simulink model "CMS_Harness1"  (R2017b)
settings: Solver=FixedStepDiscrete  StartTime=0.0  StopTime=2  FixedStep=0.01  RelTol=1e-3  EnableMultiTasking=on
undefined symbols (not defined in the file): sigbuilder_block
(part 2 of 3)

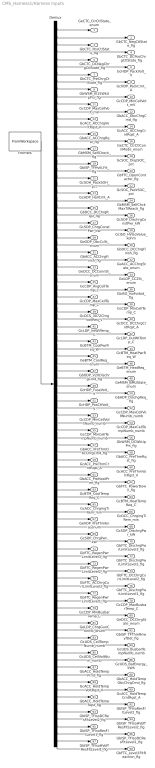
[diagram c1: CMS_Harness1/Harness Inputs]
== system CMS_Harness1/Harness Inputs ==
  Demux : Demux  Tag=STV Demux  Outputs=98
  FromWs : FromWorkspace  Tag=STV FromWs  VariableName=tuvar  SampleTime=0
  GeCTC_CtrCtlState_enum : Outport  Tag=STV Outport
  GbCTC_NegCtlState_flg : Outport  Tag=STV Outport  Port=2
  GbCTC_PosCtlState_flg : Outport  Tag=STV Outport  Port=3
  GbCTC_DCPosChrgCtlState_flg : Outport  Tag=STV Outport  Port=4
  GbCTC_DCNegChrgCtlState_flg : Outport  Tag=STV Outport  Port=5
  GcHDP_PackVolt_V : Outport  Tag=STV Outport  Port=6
  GbCTC_PreChrgCtlState_flg : Outport  Tag=STV Outport  Port=7
  GcHDP_PackCrnt_A : Outport  Tag=STV Outport  Port=8
  GbWSM_Kl15WkUpPrs_flg : Outport  Tag=STV Outport  Port=9
  GcCDP_MinCellVolt_mV : Outport  Tag=STV Outport  Port=10
  GcCDP_MaxCellVolt_mV : Outport  Tag=STV Outport  Port=11
  GbACC_ObcChrgCmd_flg : Outport  Tag=STV Outport  Port=12
  GcACC_ACChrgVoltRqst_V : Outport  Tag=STV Outport  Port=13
  GcACC_ACChrgCrntRqst_A : Outport  Tag=STV Outport  Port=14
  GbACC_ACChrgRqst_flg : Outport  Tag=STV Outport  Port=15
  GeCTC_CtrCtlConnMode_enum : Outport  Tag=STV Outport  Port=16
  GbMSM_SelfCheck_flg : Outport  Tag=STV Outport  Port=17
  GcSOC_DispSOC_pct : Outport  Tag=STV Outport  Port=18
  GbISP_TFHvilLFlt_flg : Outport  Tag=STV Outport  Port=19
  GbFTC_OpenContactor_flg : Outport  Tag=STV Outport  Port=20
  GcSOH_PackSOH_pct : Outport  Tag=STV Outport  Port=21
  GcSOC_PackSOC_pct : Outport  Tag=STV Outport  Port=22
  GcHDP_HallCrnt_A : Outport  Tag=STV Outport  Port=23
  GbMSM_SelfChckMaxTiReach_flg : Outport  Tag=STV Outport  Port=24
  GbDCC_DCChrgRqst_flg : Outport  Tag=STV Outport  Port=25
  GcSOP_DischrgConstPwr_kW : Outport  Tag=STV Outport  Port=26
  GcSOP_ChrgConstPwr_kW : Outport  Tag=STV Outport  Port=27
  GcISO_HVIsoValue_kohm : Outport  Tag=STV Outport  Port=28
  GeODP_ObcCcSt_enum : Outport  Tag=STV Outport  Port=29
  GbDCC_DCChrgFinish_flg : Outport  Tag=STV Outport  Port=30
  GbACC_ACChrgFinish_flg : Outport  Tag=STV Outport  Port=31
  GeACC_ACChrgState_enum : Outport  Tag=STV Outport  Port=32
  GeDCC_DCConnSt_enum : Outport  Tag=STV Outport  Port=33
  GeLDP_CC2St_enum : Outport  Tag=STV Outport  Port=34
  GcCDP_AvgCellTemp_C : Outport  Tag=STV Outport  Port=35
  GbISO_IsoForbid_flg : Outport  Tag=STV Outport  Port=36
  GcCDP_MaxCellTemp_C : Outport  Tag=STV Outport  Port=37
  GcCDP_MinCellTemp_C : Outport  Tag=STV Outport  Port=38
  GcDCS_3072ChrgVoltReq_V : Outport  Tag=STV Outport  Port=39
  GcDCC_DCChrgCrntRqst_A : Outport  Tag=STV Outport  Port=40
  GcLDP_lntWtTemp_C : Outport  Tag=STV Outport  Port=41
  GcLDP_OutWtTemp_C : Outport  Tag=STV Outport  Port=42
  GcBTM_CoolPwrReq_W : Outport  Tag=STV Outport  Port=43
  GcBTM_HeatPwrReq_W : Outport  Tag=STV Outport  Port=44
  GeBTM_CoolReq_enum : Outport  Tag=STV Outport  Port=45
  GeBTM_HeatReq_enum : Outport  Tag=STV Outport  Port=46
  GbODP_V2XDischrgCmd_flg : Outport  Tag=STV Outport  Port=47
  GeMSM_BMUState_enum : Outport  Tag=STV Outport  Port=48
  GcHDP_FuseVolt_V : Outport  Tag=STV Outport  Port=49
  GbADP_DischgReq_flg : Outport  Tag=STV Outport  Port=50
  GcHDP_PosCtlVolt_V : Outport  Tag=STV Outport  Port=51
  GcCDP_MaxCellVoltNumb_numb : Outport  Tag=STV Outport  Port=52
  GcCDP_MinCellVoltNumb_numb : Outport  Tag=STV Outport  Port=53
  GcCDP_MaxCellTempNumb_numb : Outport  Tag=STV Outport  Port=54
  GcCDP_MinCellTempNumb_numb : Outport  Tag=STV Outport  Port=55
  GbWSM_DCWkUpPrs_flg : Outport  Tag=STV Outport  Port=56
  GbACC_PreThmObcChrgCmd_flg : Outport  Tag=STV Outport  Port=57
  GbACC_PreThmRqst_flg : Outport  Tag=STV Outport  Port=58
  GcACC_PreThmCrntRqst_A : Outport  Tag=STV Outport  Port=59
  GcACC_PreThmVoltRqst_V : Outport  Tag=STV Outport  Port=60
  GbACC_PreHeatPrmt_flg : Outport  Tag=STV Outport  Port=61
  GbFTC_PowerDown_flg : Outport  Tag=STV Outport  Port=62
  GcBTM_CoolTempReq_C : Outport  Tag=STV Outport  Port=63
  GcBTM_HeatTempReq_C : Outport  Tag=STV Outport  Port=64
  GcACC_ChrgingTiRem_min : Outport  Tag=STV Outport  Port=65
  GcDCC_ChrgingTiRem_min : Outport  Tag=STV Outport  Port=66
  GeVDP_PreThmEna_enum : Outport  Tag=STV Outport  Port=67
  GcSOP_DischrgPwr_kW : Outport  Tag=STV Outport  Port=68
  GcSOP_ChrgPwr_kW : Outport  Tag=STV Outport  Port=69
  GbFTC_DischrgPwrLimitLevel3_flg : Outport  Tag=STV Outport  Port=70
  GbFTC_RegenPwrLimitLevel3_flg : Outport  Tag=STV Outport  Port=71
  GbFTC_DischrgPwrLimitLevel2_flg : Outport  Tag=STV Outport  Port=72
  GbFTC_RegenPwrLimitLevel2_flg : Outport  Tag=STV Outport  Port=73
  GbFTC_DCChrgCurrLimitLevel2_flg : Outport  Tag=STV Outport  Port=74
  GbFTC_ACChrgCurrLimitLevel2_flg : Outport  Tag=STV Outport  Port=75
  GbFTC_DischrgPwrLimitLevel1_flg : Outport  Tag=STV Outport  Port=76
  GbFTC_RegenPwrLimitLevel1_flg : Outport  Tag=STV Outport  Port=77
  GcCDP_MaxBusbarTemp_C : Outport  Tag=STV Outport  Port=78
  GcCDP_MinBusbarTemp_C : Outport  Tag=STV Outport  Port=79
  GeDCC_DCChrgState_enum : Outport  Tag=STV Outport  Port=80
  GeLDP_ChrgGunConnSt_enum : Outport  Tag=STV Outport  Port=81
  GbISP_TFThmRnwyfDet_flg : Outport  Tag=STV Outport  Port=82
  GcUDS_CellTempNumb_numb : Outport  Tag=STV Outport  Port=83
  GcUDS_BusbarTempNumb_numb : Outport  Tag=STV Outport  Port=84
  GcUDS_CellVoltNum_numb : Outport  Tag=STV Outport  Port=85
  GcUDS_BatEnergy_kWh : Outport  Tag=STV Outport  Port=86
  GbACC_HoldTempPrmt_flg : Outport  Tag=STV Outport  Port=87
  GbACC_HoldTempObcChrgCmd_flg : Outport  Tag=STV Outport  Port=88
  GcACC_HoldTempVoltRqst_V : Outport  Tag=STV Outport  Port=89
  GcACC_HoldTempCrntRqst_A : Outport  Tag=STV Outport  Port=90
  GbACC_HoldTempRqst_flg : Outport  Tag=STV Outport  Port=91
  GbISP_TFIsoResFltLevel2_flg : Outport  Tag=STV Outport  Port=92
  GbISP_TFIsoDCResFltLevel2_flg : Outport  Tag=STV Outport  Port=93
  GbISP_TFIsoHVoffResFltLevel2_flg : Outport  Tag=STV Outport  Port=94
  GbISP_TFIsoResFltLevel1_flg : Outport  Tag=STV Outport  Port=95
  GbISP_TFIsoDCResFltLevel1_flg : Outport  Tag=STV Outport  Port=96
  GbISP_TFIsoHVoffResFltLevel1_flg : Outport  Tag=STV Outport  Port=97
  GbFTC_Level1FltReaction_flg : Outport  Tag=STV Outport  Port=98
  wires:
  FromWs/1 -> Demux/1
  Demux/1 -> GeCTC_CtrCtlState_enum/1
  Demux/2 -> GbCTC_NegCtlState_flg/1
  Demux/3 -> GbCTC_PosCtlState_flg/1
  Demux/4 -> GbCTC_DCPosChrgCtlState_flg/1
  Demux/5 -> GbCTC_DCNegChrgCtlState_flg/1
  Demux/6 -> GcHDP_PackVolt_V/1
  Demux/7 -> GbCTC_PreChrgCtlState_flg/1
  Demux/8 -> GcHDP_PackCrnt_A/1
  Demux/9 -> GbWSM_Kl15WkUpPrs_flg/1
  Demux/10 -> GcCDP_MinCellVolt_mV/1
  Demux/11 -> GcCDP_MaxCellVolt_mV/1
  Demux/12 -> GbACC_ObcChrgCmd_flg/1
  Demux/13 -> GcACC_ACChrgVoltRqst_V/1
  Demux/14 -> GcACC_ACChrgCrntRqst_A/1
  Demux/15 -> GbACC_ACChrgRqst_flg/1
  Demux/16 -> GeCTC_CtrCtlConnMode_enum/1
  Demux/17 -> GbMSM_SelfCheck_flg/1
  Demux/18 -> GcSOC_DispSOC_pct/1
  Demux/19 -> GbISP_TFHvilLFlt_flg/1
  Demux/20 -> GbFTC_OpenContactor_flg/1
  Demux/21 -> GcSOH_PackSOH_pct/1
  Demux/22 -> GcSOC_PackSOC_pct/1
  Demux/23 -> GcHDP_HallCrnt_A/1
  Demux/24 -> GbMSM_SelfChckMaxTiReach_flg/1
  Demux/25 -> GbDCC_DCChrgRqst_flg/1
  Demux/26 -> GcSOP_DischrgConstPwr_kW/1
  Demux/27 -> GcSOP_ChrgConstPwr_kW/1
  Demux/28 -> GcISO_HVIsoValue_kohm/1
  Demux/29 -> GeODP_ObcCcSt_enum/1
  Demux/30 -> GbDCC_DCChrgFinish_flg/1
  Demux/31 -> GbACC_ACChrgFinish_flg/1
  Demux/32 -> GeACC_ACChrgState_enum/1
  Demux/33 -> GeDCC_DCConnSt_enum/1
  Demux/34 -> GeLDP_CC2St_enum/1
  Demux/35 -> GcCDP_AvgCellTemp_C/1
  Demux/36 -> GbISO_IsoForbid_flg/1
  Demux/37 -> GcCDP_MaxCellTemp_C/1
  Demux/38 -> GcCDP_MinCellTemp_C/1
  Demux/39 -> GcDCS_3072ChrgVoltReq_V/1
  Demux/40 -> GcDCC_DCChrgCrntRqst_A/1
  Demux/41 -> GcLDP_lntWtTemp_C/1
  Demux/42 -> GcLDP_OutWtTemp_C/1
  Demux/43 -> GcBTM_CoolPwrReq_W/1
  Demux/44 -> GcBTM_HeatPwrReq_W/1
  Demux/45 -> GeBTM_CoolReq_enum/1
  Demux/46 -> GeBTM_HeatReq_enum/1
  Demux/47 -> GbODP_V2XDischrgCmd_flg/1
  Demux/48 -> GeMSM_BMUState_enum/1
  Demux/49 -> GcHDP_FuseVolt_V/1
  Demux/50 -> GbADP_DischgReq_flg/1
  Demux/51 -> GcHDP_PosCtlVolt_V/1
  Demux/52 -> GcCDP_MaxCellVoltNumb_numb/1
  Demux/53 -> GcCDP_MinCellVoltNumb_numb/1
  Demux/54 -> GcCDP_MaxCellTempNumb_numb/1
  Demux/55 -> GcCDP_MinCellTempNumb_numb/1
  Demux/56 -> GbWSM_DCWkUpPrs_flg/1
  Demux/57 -> GbACC_PreThmObcChrgCmd_flg/1
  Demux/58 -> GbACC_PreThmRqst_flg/1
  Demux/59 -> GcACC_PreThmCrntRqst_A/1
  Demux/60 -> GcACC_PreThmVoltRqst_V/1
  Demux/61 -> GbACC_PreHeatPrmt_flg/1
  Demux/62 -> GbFTC_PowerDown_flg/1
  Demux/63 -> GcBTM_CoolTempReq_C/1
  Demux/64 -> GcBTM_HeatTempReq_C/1
  Demux/65 -> GcACC_ChrgingTiRem_min/1
  Demux/66 -> GcDCC_ChrgingTiRem_min/1
  Demux/67 -> GeVDP_PreThmEna_enum/1
  Demux/68 -> GcSOP_DischrgPwr_kW/1
  Demux/69 -> GcSOP_ChrgPwr_kW/1
  Demux/70 -> GbFTC_DischrgPwrLimitLevel3_flg/1
  Demux/71 -> GbFTC_RegenPwrLimitLevel3_flg/1
  Demux/72 -> GbFTC_DischrgPwrLimitLevel2_flg/1
  Demux/73 -> GbFTC_RegenPwrLimitLevel2_flg/1
  Demux/74 -> GbFTC_DCChrgCurrLimitLevel2_flg/1
  Demux/75 -> GbFTC_ACChrgCurrLimitLevel2_flg/1
  Demux/76 -> GbFTC_DischrgPwrLimitLevel1_flg/1
  Demux/77 -> GbFTC_RegenPwrLimitLevel1_flg/1
  Demux/78 -> GcCDP_MaxBusbarTemp_C/1
  Demux/79 -> GcCDP_MinBusbarTemp_C/1
  Demux/80 -> GeDCC_DCChrgState_enum/1
  Demux/81 -> GeLDP_ChrgGunConnSt_enum/1
  Demux/82 -> GbISP_TFThmRnwyfDet_flg/1
  Demux/83 -> GcUDS_CellTempNumb_numb/1
  Demux/84 -> GcUDS_BusbarTempNumb_numb/1
  Demux/85 -> GcUDS_CellVoltNum_numb/1
  Demux/86 -> GcUDS_BatEnergy_kWh/1
  Demux/87 -> GbACC_HoldTempPrmt_flg/1
  Demux/88 -> GbACC_HoldTempObcChrgCmd_flg/1
  Demux/89 -> GcACC_HoldTempVoltRqst_V/1
  Demux/90 -> GcACC_HoldTempCrntRqst_A/1
  Demux/91 -> GbACC_HoldTempRqst_flg/1
  Demux/92 -> GbISP_TFIsoResFltLevel2_flg/1
  Demux/93 -> GbISP_TFIsoDCResFltLevel2_flg/1
  Demux/94 -> GbISP_TFIsoHVoffResFltLevel2_flg/1
  Demux/95 -> GbISP_TFIsoResFltLevel1_flg/1
  Demux/96 -> GbISP_TFIsoDCResFltLevel1_flg/1
  Demux/97 -> GbISP_TFIsoHVoffResFltLevel1_flg/1
  Demux/98 -> GbFTC_Level1FltReaction_flg/1

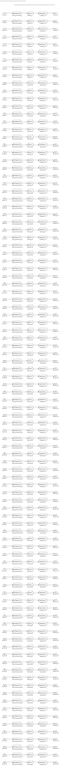
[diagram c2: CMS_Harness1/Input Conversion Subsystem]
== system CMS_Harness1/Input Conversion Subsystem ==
  note: This subsystem has been inserted by Simulink to adapt the output of the source blocks to the interface required by the harnessed component. Modifying the contents of this subsystem may result in compilation and simulation failure.
  Inport_1 : Inport
  Inport_2 : Inport  Port=2
  Inport_3 : Inport  Port=3
  Inport_4 : Inport  Port=4
  Inport_5 : Inport  Port=5
  Inport_6 : Inport  Port=6
  Inport_7 : Inport  Port=7
  Inport_8 : Inport  Port=8
  Inport_9 : Inport  Port=9
  Inport_10 : Inport  Port=10
  Inport_11 : Inport  Port=11
  Inport_12 : Inport  Port=12
  Inport_13 : Inport  Port=13
  Inport_14 : Inport  Port=14
  Inport_15 : Inport  Port=15
  Inport_16 : Inport  Port=16
  Inport_17 : Inport  Port=17
  Inport_18 : Inport  Port=18
  Inport_19 : Inport  Port=19
  Inport_20 : Inport  Port=20
  Inport_21 : Inport  Port=21
  Inport_22 : Inport  Port=22
  Inport_23 : Inport  Port=23
  Inport_24 : Inport  Port=24
  Inport_25 : Inport  Port=25
  Inport_26 : Inport  Port=26
  Inport_27 : Inport  Port=27
  Inport_28 : Inport  Port=28
  Inport_29 : Inport  Port=29
  Inport_30 : Inport  Port=30
  Inport_31 : Inport  Port=31
  Inport_32 : Inport  Port=32
  Inport_33 : Inport  Port=33
  Inport_34 : Inport  Port=34
  Inport_35 : Inport  Port=35
  Inport_36 : Inport  Port=36
  Inport_37 : Inport  Port=37
  Inport_38 : Inport  Port=38
  Inport_39 : Inport  Port=39
  Inport_40 : Inport  Port=40
  Inport_41 : Inport  Port=41
  Inport_42 : Inport  Port=42
  Inport_43 : Inport  Port=43
  Inport_44 : Inport  Port=44
  Inport_45 : Inport  Port=45
  Inport_46 : Inport  Port=46
  Inport_47 : Inport  Port=47
  Inport_48 : Inport  Port=48
  Inport_49 : Inport  Port=49
  Inport_50 : Inport  Port=50
  Inport_51 : Inport  Port=51
  Inport_52 : Inport  Port=52
  Inport_53 : Inport  Port=53
  Inport_54 : Inport  Port=54
  Inport_55 : Inport  Port=55
  Inport_56 : Inport  Port=56
  Inport_57 : Inport  Port=57
  Inport_58 : Inport  Port=58
  Inport_59 : Inport  Port=59
  Inport_60 : Inport  Port=60
  Inport_61 : Inport  Port=61
  Inport_62 : Inport  Port=62
  Inport_63 : Inport  Port=63
  Inport_64 : Inport  Port=64
  Inport_65 : Inport  Port=65
  Inport_66 : Inport  Port=66
  Inport_67 : Inport  Port=67
  Inport_68 : Inport  Port=68
  Inport_69 : Inport  Port=69
  Inport_70 : Inport  Port=70
  Inport_71 : Inport  Port=71
  Inport_72 : Inport  Port=72
  Inport_73 : Inport  Port=73
  Inport_74 : Inport  Port=74
  Inport_75 : Inport  Port=75
  Inport_76 : Inport  Port=76
  Inport_77 : Inport  Port=77
  Inport_78 : Inport  Port=78
  Inport_79 : Inport  Port=79
  Inport_80 : Inport  Port=80
  Inport_81 : Inport  Port=81
  Inport_82 : Inport  Port=82
  Inport_83 : Inport  Port=83
  Inport_84 : Inport  Port=84
  Inport_85 : Inport  Port=85
  Inport_86 : Inport  Port=86
  Inport_87 : Inport  Port=87
  Inport_88 : Inport  Port=88
  Inport_89 : Inport  Port=89
  Inport_90 : Inport  Port=90
  Inport_91 : Inport  Port=91
  Inport_92 : Inport  Port=92
  Inport_93 : Inport  Port=93
  Inport_94 : Inport  Port=94
  Inport_95 : Inport  Port=95
  Inport_96 : Inport  Port=96
  Inport_97 : Inport  Port=97
  Inport_98 : Inport  Port=98
  Data_Conversion_{1,16,29,32..34,45..46,48,52..55,67,80..81,83..85} (19 alike) : DataTypeConversion  OutDataTypeStr=uint8
  Data_Conversion_{10..11,28,65..66,86} (6 alike) : DataTypeConversion  OutDataTypeStr=uint16
  Data_Conversion_{2..5,7,9,12,15,17,19..20,24..25,30..31,36,47,50,56..58,61..62,70..77,82,87..88,91..98} (42 alike) : DataTypeConversion  OutDataTypeStr=boolean
  Data_Conversion_{6,8,13..14,18,21..23,26..27,35,37..38,40..44,49,51,59..60,63..64,68..69,78..79,89..90} (30 alike) : DataTypeConversion  OutDataTypeStr=single
  Data_Conversion_39 : DataTypeConversion  OutDataTypeStr=fixdt('ufix16_Sp1')
  RateTs_{1..98} (98 alike) : RateTransition  OutPortSampleTime=0.01
  SigSpec_{1,16,32..34,45..46,48,67,80} (10 alike) : SignalSpecification  OutDataTypeStr=uint8  Unit=enum  Dimensions=[1]  SampleTime=0.01
  SigSpec_10 : SignalSpecification  OutDataTypeStr=uint16  Unit=mV  Dimensions=[1]  SampleTime=0.01
  SigSpec_11 : SignalSpecification  OutDataTypeStr=uint16  Unit=mV  Dimensions=[1]  SampleTime=0.01
  SigSpec_{12,15,17,19..20,24..25,30..31,36,47,57..58,61..62,70..77,82,87..88,91..98} (34 alike) : SignalSpecification  OutDataTypeStr=boolean  Unit=flag  Dimensions=[1]  SampleTime=0.01
  SigSpec_{6,13,49,51,60,89} (6 alike) : SignalSpecification  OutDataTypeStr=single  Unit=V  Dimensions=[1]  SampleTime=0.01
  SigSpec_{8,14,23,40,59,90} (6 alike) : SignalSpecification  OutDataTypeStr=single  Unit=A  Dimensions=[1]  SampleTime=0.01
  SigSpec_18 : SignalSpecification  OutDataTypeStr=single  Unit=pct  Dimensions=[1]  SampleTime=0.01
  SigSpec_{2..5,7,9,50,56} (8 alike) : SignalSpecification  OutDataTypeStr=boolean  Unit=flg  Dimensions=[1]  SampleTime=0.01
  SigSpec_21 : SignalSpecification  OutDataTypeStr=single  Unit=pct  Dimensions=[1]  SampleTime=0.01
  SigSpec_22 : SignalSpecification  OutDataTypeStr=single  Unit=pct  Dimensions=[1]  SampleTime=0.01
  SigSpec_{26..27,68..69} (4 alike) : SignalSpecification  OutDataTypeStr=single  Unit=kW  Dimensions=[1]  SampleTime=0.01
  SigSpec_28 : SignalSpecification  OutDataTypeStr=uint16  Unit=kohm  Dimensions=[1]  SampleTime=0.01
  SigSpec_{29,52..55,81,83..85} (9 alike) : SignalSpecification  OutDataTypeStr=uint8  Unit=numb  Dimensions=[1]  SampleTime=0.01
  SigSpec_{35,37..38,41..42,63..64,78..79} (9 alike) : SignalSpecification  OutDataTypeStr=single  Unit=C  Dimensions=[1]  SampleTime=0.01
  SigSpec_39 : SignalSpecification  OutDataTypeStr=fixdt('ufix16_Sp1')  Unit=V  Dimensions=[1]  SampleTime=0.01
  SigSpec_43 : SignalSpecification  OutDataTypeStr=single  Unit=W  Dimensions=[1]  SampleTime=0.01
  SigSpec_44 : SignalSpecification  OutDataTypeStr=single  Unit=W  Dimensions=[1]  SampleTime=0.01
  SigSpec_65 : SignalSpecification  OutDataTypeStr=uint16  Unit=min  Dimensions=[1]  SampleTime=0.01
  SigSpec_66 : SignalSpecification  OutDataTypeStr=uint16  Unit=min  Dimensions=[1]  SampleTime=0.01
  SigSpec_86 : SignalSpecification  OutDataTypeStr=uint16  Unit=kWh  Dimensions=[1]  SampleTime=0.01
  Outport_1 : Outport
  Outport_2 : Outport  Port=2
  Outport_3 : Outport  Port=3
  Outport_4 : Outport  Port=4
  Outport_5 : Outport  Port=5
  Outport_6 : Outport  Port=6
  Outport_7 : Outport  Port=7
  Outport_8 : Outport  Port=8
  Outport_9 : Outport  Port=9
  Outport_10 : Outport  Port=10
  Outport_11 : Outport  Port=11
  Outport_12 : Outport  Port=12
  Outport_13 : Outport  Port=13
  Outport_14 : Outport  Port=14
  Outport_15 : Outport  Port=15
  Outport_16 : Outport  Port=16
  Outport_17 : Outport  Port=17
  Outport_18 : Outport  Port=18
  Outport_19 : Outport  Port=19
  Outport_20 : Outport  Port=20
  Outport_21 : Outport  Port=21
  Outport_22 : Outport  Port=22
  Outport_23 : Outport  Port=23
  Outport_24 : Outport  Port=24
  Outport_25 : Outport  Port=25
  Outport_26 : Outport  Port=26
  Outport_27 : Outport  Port=27
  Outport_28 : Outport  Port=28
  Outport_29 : Outport  Port=29
  Outport_30 : Outport  Port=30
  Outport_31 : Outport  Port=31
  Outport_32 : Outport  Port=32
  Outport_33 : Outport  Port=33
  Outport_34 : Outport  Port=34
  Outport_35 : Outport  Port=35
  Outport_36 : Outport  Port=36
  Outport_37 : Outport  Port=37
  Outport_38 : Outport  Port=38
  Outport_39 : Outport  Port=39
  Outport_40 : Outport  Port=40
  Outport_41 : Outport  Port=41
  Outport_42 : Outport  Port=42
  Outport_43 : Outport  Port=43
  Outport_44 : Outport  Port=44
  Outport_45 : Outport  Port=45
  Outport_46 : Outport  Port=46
  Outport_47 : Outport  Port=47
  Outport_48 : Outport  Port=48
  Outport_49 : Outport  Port=49
  Outport_50 : Outport  Port=50
  Outport_51 : Outport  Port=51
  Outport_52 : Outport  Port=52
  Outport_53 : Outport  Port=53
  Outport_54 : Outport  Port=54
  Outport_55 : Outport  Port=55
  Outport_56 : Outport  Port=56
  Outport_57 : Outport  Port=57
  Outport_58 : Outport  Port=58
  Outport_59 : Outport  Port=59
  Outport_60 : Outport  Port=60
  Outport_61 : Outport  Port=61
  Outport_62 : Outport  Port=62
  Outport_63 : Outport  Port=63
  Outport_64 : Outport  Port=64
  Outport_65 : Outport  Port=65
  Outport_66 : Outport  Port=66
  Outport_67 : Outport  Port=67
  Outport_68 : Outport  Port=68
  Outport_69 : Outport  Port=69
  Outport_70 : Outport  Port=70
  Outport_71 : Outport  Port=71
  Outport_72 : Outport  Port=72
  Outport_73 : Outport  Port=73
  Outport_74 : Outport  Port=74
  Outport_75 : Outport  Port=75
  Outport_76 : Outport  Port=76
  Outport_77 : Outport  Port=77
  Outport_78 : Outport  Port=78
  Outport_79 : Outport  Port=79
  Outport_80 : Outport  Port=80
  Outport_81 : Outport  Port=81
  Outport_82 : Outport  Port=82
  Outport_83 : Outport  Port=83
  Outport_84 : Outport  Port=84
  Outport_85 : Outport  Port=85
  Outport_86 : Outport  Port=86
  Outport_87 : Outport  Port=87
  Outport_88 : Outport  Port=88
  Outport_89 : Outport  Port=89
  Outport_90 : Outport  Port=90
  Outport_91 : Outport  Port=91
  Outport_92 : Outport  Port=92
  Outport_93 : Outport  Port=93
  Outport_94 : Outport  Port=94
  Outport_95 : Outport  Port=95
  Outport_96 : Outport  Port=96
  Outport_97 : Outport  Port=97
  Outport_98 : Outport  Port=98
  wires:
  SigSpec_1/1 -> Outport_1/1
  RateTs_1/1 -> SigSpec_1/1
  Data_Conversion_1/1 -> RateTs_1/1
  Inport_1/1 -> Data_Conversion_1/1
  SigSpec_2/1 -> Outport_2/1
  RateTs_2/1 -> SigSpec_2/1
  Data_Conversion_2/1 -> RateTs_2/1
  Inport_2/1 -> Data_Conversion_2/1
  SigSpec_3/1 -> Outport_3/1
  RateTs_3/1 -> SigSpec_3/1
  Data_Conversion_3/1 -> RateTs_3/1
  Inport_3/1 -> Data_Conversion_3/1
  SigSpec_4/1 -> Outport_4/1
  RateTs_4/1 -> SigSpec_4/1
  Data_Conversion_4/1 -> RateTs_4/1
  Inport_4/1 -> Data_Conversion_4/1
  SigSpec_5/1 -> Outport_5/1
  RateTs_5/1 -> SigSpec_5/1
  Data_Conversion_5/1 -> RateTs_5/1
  Inport_5/1 -> Data_Conversion_5/1
  SigSpec_6/1 -> Outport_6/1
  RateTs_6/1 -> SigSpec_6/1
  Data_Conversion_6/1 -> RateTs_6/1
  Inport_6/1 -> Data_Conversion_6/1
  SigSpec_7/1 -> Outport_7/1
  RateTs_7/1 -> SigSpec_7/1
  Data_Conversion_7/1 -> RateTs_7/1
  Inport_7/1 -> Data_Conversion_7/1
  SigSpec_8/1 -> Outport_8/1
  RateTs_8/1 -> SigSpec_8/1
  Data_Conversion_8/1 -> RateTs_8/1
  Inport_8/1 -> Data_Conversion_8/1
  SigSpec_9/1 -> Outport_9/1
  RateTs_9/1 -> SigSpec_9/1
  Data_Conversion_9/1 -> RateTs_9/1
  Inport_9/1 -> Data_Conversion_9/1
  SigSpec_10/1 -> Outport_10/1
  RateTs_10/1 -> SigSpec_10/1
  Data_Conversion_10/1 -> RateTs_10/1
  Inport_10/1 -> Data_Conversion_10/1
  SigSpec_11/1 -> Outport_11/1
  RateTs_11/1 -> SigSpec_11/1
  Data_Conversion_11/1 -> RateTs_11/1
  Inport_11/1 -> Data_Conversion_11/1
  SigSpec_12/1 -> Outport_12/1
  RateTs_12/1 -> SigSpec_12/1
  Data_Conversion_12/1 -> RateTs_12/1
  Inport_12/1 -> Data_Conversion_12/1
  SigSpec_13/1 -> Outport_13/1
  RateTs_13/1 -> SigSpec_13/1
  Data_Conversion_13/1 -> RateTs_13/1
  Inport_13/1 -> Data_Conversion_13/1
  SigSpec_14/1 -> Outport_14/1
  RateTs_14/1 -> SigSpec_14/1
  Data_Conversion_14/1 -> RateTs_14/1
  Inport_14/1 -> Data_Conversion_14/1
  SigSpec_15/1 -> Outport_15/1
  RateTs_15/1 -> SigSpec_15/1
  Data_Conversion_15/1 -> RateTs_15/1
  Inport_15/1 -> Data_Conversion_15/1
  SigSpec_16/1 -> Outport_16/1
  RateTs_16/1 -> SigSpec_16/1
  Data_Conversion_16/1 -> RateTs_16/1
  Inport_16/1 -> Data_Conversion_16/1
  SigSpec_17/1 -> Outport_17/1
  RateTs_17/1 -> SigSpec_17/1
  Data_Conversion_17/1 -> RateTs_17/1
  Inport_17/1 -> Data_Conversion_17/1
  SigSpec_18/1 -> Outport_18/1
  RateTs_18/1 -> SigSpec_18/1
  Data_Conversion_18/1 -> RateTs_18/1
  Inport_18/1 -> Data_Conversion_18/1
  SigSpec_19/1 -> Outport_19/1
  RateTs_19/1 -> SigSpec_19/1
  Data_Conversion_19/1 -> RateTs_19/1
  Inport_19/1 -> Data_Conversion_19/1
  SigSpec_20/1 -> Outport_20/1
  RateTs_20/1 -> SigSpec_20/1
  Data_Conversion_20/1 -> RateTs_20/1
  Inport_20/1 -> Data_Conversion_20/1
  SigSpec_21/1 -> Outport_21/1
  RateTs_21/1 -> SigSpec_21/1
  Data_Conversion_21/1 -> RateTs_21/1
  Inport_21/1 -> Data_Conversion_21/1
  SigSpec_22/1 -> Outport_22/1
  RateTs_22/1 -> SigSpec_22/1
  Data_Conversion_22/1 -> RateTs_22/1
  Inport_22/1 -> Data_Conversion_22/1
  SigSpec_23/1 -> Outport_23/1
  RateTs_23/1 -> SigSpec_23/1
  Data_Conversion_23/1 -> RateTs_23/1
  Inport_23/1 -> Data_Conversion_23/1
  SigSpec_24/1 -> Outport_24/1
  RateTs_24/1 -> SigSpec_24/1
  Data_Conversion_24/1 -> RateTs_24/1
  Inport_24/1 -> Data_Conversion_24/1
  SigSpec_25/1 -> Outport_25/1
  RateTs_25/1 -> SigSpec_25/1
  Data_Conversion_25/1 -> RateTs_25/1
  Inport_25/1 -> Data_Conversion_25/1
  SigSpec_26/1 -> Outport_26/1
  RateTs_26/1 -> SigSpec_26/1
  Data_Conversion_26/1 -> RateTs_26/1
  Inport_26/1 -> Data_Conversion_26/1
  SigSpec_27/1 -> Outport_27/1
  RateTs_27/1 -> SigSpec_27/1
  Data_Conversion_27/1 -> RateTs_27/1
  Inport_27/1 -> Data_Conversion_27/1
  SigSpec_28/1 -> Outport_28/1
  RateTs_28/1 -> SigSpec_28/1
  Data_Conversion_28/1 -> RateTs_28/1
  Inport_28/1 -> Data_Conversion_28/1
  SigSpec_29/1 -> Outport_29/1
  RateTs_29/1 -> SigSpec_29/1
  Data_Conversion_29/1 -> RateTs_29/1
  Inport_29/1 -> Data_Conversion_29/1
  SigSpec_30/1 -> Outport_30/1
  RateTs_30/1 -> SigSpec_30/1
  Data_Conversion_30/1 -> RateTs_30/1
  Inport_30/1 -> Data_Conversion_30/1
  SigSpec_31/1 -> Outport_31/1
  RateTs_31/1 -> SigSpec_31/1
  Data_Conversion_31/1 -> RateTs_31/1
  Inport_31/1 -> Data_Conversion_31/1
  SigSpec_32/1 -> Outport_32/1
  RateTs_32/1 -> SigSpec_32/1
  Data_Conversion_32/1 -> RateTs_32/1
  Inport_32/1 -> Data_Conversion_32/1
  SigSpec_33/1 -> Outport_33/1
  RateTs_33/1 -> SigSpec_33/1
  Data_Conversion_33/1 -> RateTs_33/1
  Inport_33/1 -> Data_Conversion_33/1
  SigSpec_34/1 -> Outport_34/1
  RateTs_34/1 -> SigSpec_34/1
  Data_Conversion_34/1 -> RateTs_34/1
  Inport_34/1 -> Data_Conversion_34/1
  SigSpec_35/1 -> Outport_35/1
  RateTs_35/1 -> SigSpec_35/1
  Data_Conversion_35/1 -> RateTs_35/1
  Inport_35/1 -> Data_Conversion_35/1
  SigSpec_36/1 -> Outport_36/1
  RateTs_36/1 -> SigSpec_36/1
  Data_Conversion_36/1 -> RateTs_36/1
  Inport_36/1 -> Data_Conversion_36/1
  SigSpec_37/1 -> Outport_37/1
  RateTs_37/1 -> SigSpec_37/1
  Data_Conversion_37/1 -> RateTs_37/1
  Inport_37/1 -> Data_Conversion_37/1
  SigSpec_38/1 -> Outport_38/1
  RateTs_38/1 -> SigSpec_38/1
  Data_Conversion_38/1 -> RateTs_38/1
  Inport_38/1 -> Data_Conversion_38/1
  SigSpec_39/1 -> Outport_39/1
  RateTs_39/1 -> SigSpec_39/1
  Data_Conversion_39/1 -> RateTs_39/1
  Inport_39/1 -> Data_Conversion_39/1
  SigSpec_40/1 -> Outport_40/1
  RateTs_40/1 -> SigSpec_40/1
  Data_Conversion_40/1 -> RateTs_40/1
  Inport_40/1 -> Data_Conversion_40/1
  SigSpec_41/1 -> Outport_41/1
  RateTs_41/1 -> SigSpec_41/1
  Data_Conversion_41/1 -> RateTs_41/1
  Inport_41/1 -> Data_Conversion_41/1
  SigSpec_42/1 -> Outport_42/1
  RateTs_42/1 -> SigSpec_42/1
  Data_Conversion_42/1 -> RateTs_42/1
  Inport_42/1 -> Data_Conversion_42/1
  SigSpec_43/1 -> Outport_43/1
  RateTs_43/1 -> SigSpec_43/1
  Data_Conversion_43/1 -> RateTs_43/1
  Inport_43/1 -> Data_Conversion_43/1
  SigSpec_44/1 -> Outport_44/1
  RateTs_44/1 -> SigSpec_44/1
  Data_Conversion_44/1 -> RateTs_44/1
  Inport_44/1 -> Data_Conversion_44/1
  SigSpec_45/1 -> Outport_45/1
  RateTs_45/1 -> SigSpec_45/1
  Data_Conversion_45/1 -> RateTs_45/1
  Inport_45/1 -> Data_Conversion_45/1
  SigSpec_46/1 -> Outport_46/1
  RateTs_46/1 -> SigSpec_46/1
  Data_Conversion_46/1 -> RateTs_46/1
  Inport_46/1 -> Data_Conversion_46/1
  SigSpec_47/1 -> Outport_47/1
  RateTs_47/1 -> SigSpec_47/1
  Data_Conversion_47/1 -> RateTs_47/1
  Inport_47/1 -> Data_Conversion_47/1
  SigSpec_48/1 -> Outport_48/1
  RateTs_48/1 -> SigSpec_48/1
  Data_Conversion_48/1 -> RateTs_48/1
  Inport_48/1 -> Data_Conversion_48/1
  SigSpec_49/1 -> Outport_49/1
  RateTs_49/1 -> SigSpec_49/1
  Data_Conversion_49/1 -> RateTs_49/1
  Inport_49/1 -> Data_Conversion_49/1
  SigSpec_50/1 -> Outport_50/1
  RateTs_50/1 -> SigSpec_50/1
  Data_Conversion_50/1 -> RateTs_50/1
  Inport_50/1 -> Data_Conversion_50/1
  SigSpec_51/1 -> Outport_51/1
  RateTs_51/1 -> SigSpec_51/1
  Data_Conversion_51/1 -> RateTs_51/1
  Inport_51/1 -> Data_Conversion_51/1
  SigSpec_52/1 -> Outport_52/1
  RateTs_52/1 -> SigSpec_52/1
  Data_Conversion_52/1 -> RateTs_52/1
  Inport_52/1 -> Data_Conversion_52/1
  SigSpec_53/1 -> Outport_53/1
  RateTs_53/1 -> SigSpec_53/1
  Data_Conversion_53/1 -> RateTs_53/1
  Inport_53/1 -> Data_Conversion_53/1
  SigSpec_54/1 -> Outport_54/1
  RateTs_54/1 -> SigSpec_54/1
  Data_Conversion_54/1 -> RateTs_54/1
  Inport_54/1 -> Data_Conversion_54/1
  SigSpec_55/1 -> Outport_55/1
  RateTs_55/1 -> SigSpec_55/1
  Data_Conversion_55/1 -> RateTs_55/1
  Inport_55/1 -> Data_Conversion_55/1
  SigSpec_56/1 -> Outport_56/1
  RateTs_56/1 -> SigSpec_56/1
  Data_Conversion_56/1 -> RateTs_56/1
  Inport_56/1 -> Data_Conversion_56/1
  SigSpec_57/1 -> Outport_57/1
  RateTs_57/1 -> SigSpec_57/1
  Data_Conversion_57/1 -> RateTs_57/1
  Inport_57/1 -> Data_Conversion_57/1
  SigSpec_58/1 -> Outport_58/1
  RateTs_58/1 -> SigSpec_58/1
  Data_Conversion_58/1 -> RateTs_58/1
  Inport_58/1 -> Data_Conversion_58/1
  SigSpec_59/1 -> Outport_59/1
  RateTs_59/1 -> SigSpec_59/1
  Data_Conversion_59/1 -> RateTs_59/1
  Inport_59/1 -> Data_Conversion_59/1
  SigSpec_60/1 -> Outport_60/1
  RateTs_60/1 -> SigSpec_60/1
  Data_Conversion_60/1 -> RateTs_60/1
  Inport_60/1 -> Data_Conversion_60/1
  SigSpec_61/1 -> Outport_61/1
  RateTs_61/1 -> SigSpec_61/1
  Data_Conversion_61/1 -> RateTs_61/1
  Inport_61/1 -> Data_Conversion_61/1
  SigSpec_62/1 -> Outport_62/1
  RateTs_62/1 -> SigSpec_62/1
  Data_Conversion_62/1 -> RateTs_62/1
  Inport_62/1 -> Data_Conversion_62/1
  SigSpec_63/1 -> Outport_63/1
  RateTs_63/1 -> SigSpec_63/1
  Data_Conversion_63/1 -> RateTs_63/1
  Inport_63/1 -> Data_Conversion_63/1
  SigSpec_64/1 -> Outport_64/1
  RateTs_64/1 -> SigSpec_64/1
  Data_Conversion_64/1 -> RateTs_64/1
  Inport_64/1 -> Data_Conversion_64/1
  SigSpec_65/1 -> Outport_65/1
  RateTs_65/1 -> SigSpec_65/1
  Data_Conversion_65/1 -> RateTs_65/1
  Inport_65/1 -> Data_Conversion_65/1
  SigSpec_66/1 -> Outport_66/1
  RateTs_66/1 -> SigSpec_66/1
  Data_Conversion_66/1 -> RateTs_66/1
  Inport_66/1 -> Data_Conversion_66/1
  SigSpec_67/1 -> Outport_67/1
  RateTs_67/1 -> SigSpec_67/1
  Data_Conversion_67/1 -> RateTs_67/1
  Inport_67/1 -> Data_Conversion_67/1
  SigSpec_68/1 -> Outport_68/1
  RateTs_68/1 -> SigSpec_68/1
  Data_Conversion_68/1 -> RateTs_68/1
  Inport_68/1 -> Data_Conversion_68/1
  SigSpec_69/1 -> Outport_69/1
  RateTs_69/1 -> SigSpec_69/1
  Data_Conversion_69/1 -> RateTs_69/1
  Inport_69/1 -> Data_Conversion_69/1
  SigSpec_70/1 -> Outport_70/1
  RateTs_70/1 -> SigSpec_70/1
  Data_Conversion_70/1 -> RateTs_70/1
  Inport_70/1 -> Data_Conversion_70/1
  SigSpec_71/1 -> Outport_71/1
  RateTs_71/1 -> SigSpec_71/1
  Data_Conversion_71/1 -> RateTs_71/1
  Inport_71/1 -> Data_Conversion_71/1
  SigSpec_72/1 -> Outport_72/1
  RateTs_72/1 -> SigSpec_72/1
  Data_Conversion_72/1 -> RateTs_72/1
  Inport_72/1 -> Data_Conversion_72/1
  SigSpec_73/1 -> Outport_73/1
  RateTs_73/1 -> SigSpec_73/1
  Data_Conversion_73/1 -> RateTs_73/1
  Inport_73/1 -> Data_Conversion_73/1
  SigSpec_74/1 -> Outport_74/1
  RateTs_74/1 -> SigSpec_74/1
  Data_Conversion_74/1 -> RateTs_74/1
  Inport_74/1 -> Data_Conversion_74/1
  SigSpec_75/1 -> Outport_75/1
  RateTs_75/1 -> SigSpec_75/1
  Data_Conversion_75/1 -> RateTs_75/1
  Inport_75/1 -> Data_Conversion_75/1
  SigSpec_76/1 -> Outport_76/1
  RateTs_76/1 -> SigSpec_76/1
  Data_Conversion_76/1 -> RateTs_76/1
  Inport_76/1 -> Data_Conversion_76/1
  SigSpec_77/1 -> Outport_77/1
  RateTs_77/1 -> SigSpec_77/1
  Data_Conversion_77/1 -> RateTs_77/1
  Inport_77/1 -> Data_Conversion_77/1
  SigSpec_78/1 -> Outport_78/1
  RateTs_78/1 -> SigSpec_78/1
  Data_Conversion_78/1 -> RateTs_78/1
  Inport_78/1 -> Data_Conversion_78/1
  SigSpec_79/1 -> Outport_79/1
  RateTs_79/1 -> SigSpec_79/1
  Data_Conversion_79/1 -> RateTs_79/1
  Inport_79/1 -> Data_Conversion_79/1
  SigSpec_80/1 -> Outport_80/1
  RateTs_80/1 -> SigSpec_80/1
  Data_Conversion_80/1 -> RateTs_80/1
  Inport_80/1 -> Data_Conversion_80/1
  SigSpec_81/1 -> Outport_81/1
  RateTs_81/1 -> SigSpec_81/1
  Data_Conversion_81/1 -> RateTs_81/1
  Inport_81/1 -> Data_Conversion_81/1
  SigSpec_82/1 -> Outport_82/1
  RateTs_82/1 -> SigSpec_82/1
  Data_Conversion_82/1 -> RateTs_82/1
  Inport_82/1 -> Data_Conversion_82/1
  SigSpec_83/1 -> Outport_83/1
  RateTs_83/1 -> SigSpec_83/1
  Data_Conversion_83/1 -> RateTs_83/1
  Inport_83/1 -> Data_Conversion_83/1
  SigSpec_84/1 -> Outport_84/1
  RateTs_84/1 -> SigSpec_84/1
  Data_Conversion_84/1 -> RateTs_84/1
  Inport_84/1 -> Data_Conversion_84/1
  SigSpec_85/1 -> Outport_85/1
  RateTs_85/1 -> SigSpec_85/1
  Data_Conversion_85/1 -> RateTs_85/1
  Inport_85/1 -> Data_Conversion_85/1
  SigSpec_86/1 -> Outport_86/1
  RateTs_86/1 -> SigSpec_86/1
  Data_Conversion_86/1 -> RateTs_86/1
  Inport_86/1 -> Data_Conversion_86/1
  SigSpec_87/1 -> Outport_87/1
  RateTs_87/1 -> SigSpec_87/1
  Data_Conversion_87/1 -> RateTs_87/1
  Inport_87/1 -> Data_Conversion_87/1
  SigSpec_88/1 -> Outport_88/1
  RateTs_88/1 -> SigSpec_88/1
  Data_Conversion_88/1 -> RateTs_88/1
  Inport_88/1 -> Data_Conversion_88/1
  SigSpec_89/1 -> Outport_89/1
  RateTs_89/1 -> SigSpec_89/1
  Data_Conversion_89/1 -> RateTs_89/1
  Inport_89/1 -> Data_Conversion_89/1
  SigSpec_90/1 -> Outport_90/1
  RateTs_90/1 -> SigSpec_90/1
  Data_Conversion_90/1 -> RateTs_90/1
  Inport_90/1 -> Data_Conversion_90/1
  SigSpec_91/1 -> Outport_91/1
  RateTs_91/1 -> SigSpec_91/1
  Data_Conversion_91/1 -> RateTs_91/1
  Inport_91/1 -> Data_Conversion_91/1
  SigSpec_92/1 -> Outport_92/1
  RateTs_92/1 -> SigSpec_92/1
  Data_Conversion_92/1 -> RateTs_92/1
  Inport_92/1 -> Data_Conversion_92/1
  SigSpec_93/1 -> Outport_93/1
  RateTs_93/1 -> SigSpec_93/1
  Data_Conversion_93/1 -> RateTs_93/1
  Inport_93/1 -> Data_Conversion_93/1
  SigSpec_94/1 -> Outport_94/1
  RateTs_94/1 -> SigSpec_94/1
  Data_Conversion_94/1 -> RateTs_94/1
  Inport_94/1 -> Data_Conversion_94/1
  SigSpec_95/1 -> Outport_95/1
  RateTs_95/1 -> SigSpec_95/1
  Data_Conversion_95/1 -> RateTs_95/1
  Inport_95/1 -> Data_Conversion_95/1
  SigSpec_96/1 -> Outport_96/1
  RateTs_96/1 -> SigSpec_96/1
  Data_Conversion_96/1 -> RateTs_96/1
  Inport_96/1 -> Data_Conversion_96/1
  SigSpec_97/1 -> Outport_97/1
  RateTs_97/1 -> SigSpec_97/1
  Data_Conversion_97/1 -> RateTs_97/1
  Inport_97/1 -> Data_Conversion_97/1
  SigSpec_98/1 -> Outport_98/1
  RateTs_98/1 -> SigSpec_98/1
  Data_Conversion_98/1 -> RateTs_98/1
  Inport_98/1 -> Data_Conversion_98/1
